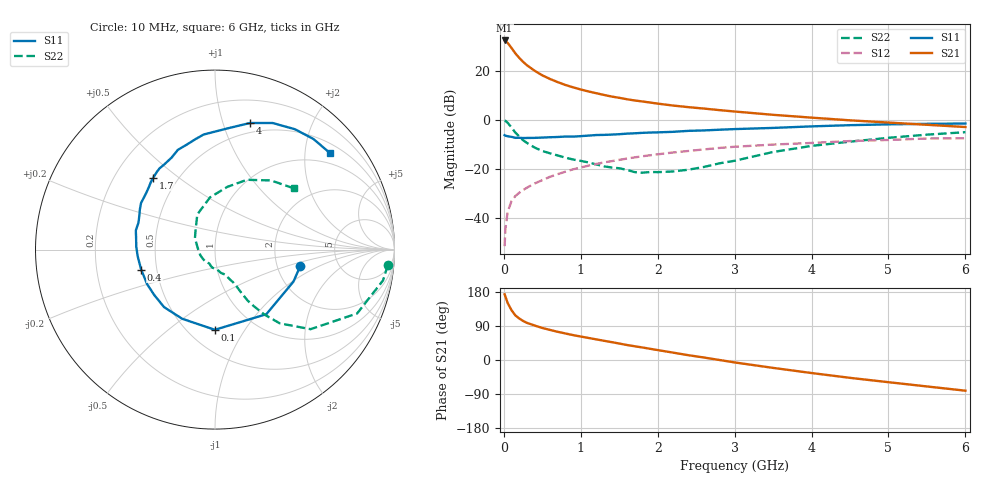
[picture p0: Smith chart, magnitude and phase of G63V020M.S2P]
! SIEMENS Small Signal Semiconductors
! BFG193
! Si NPN RF Bipolar Junction Transistor in SOT223
! VCE = 3 V  IC = 20 mA
! Common Emitter S-Parameters:  August  1996
# GHz  S  MA  R  50
!  f  S11  S21  S12  S22
! GHz  MAG  ANG  MAG  ANG  MAG  ANG  MAG  ANG
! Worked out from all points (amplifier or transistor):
!   36 points, 10 MHz to 6 GHz, reference 50 ohm
!   highest |S21| = 32.4 dB at 10 MHz (marker M1)
!   |S21| within 3 dB of that: start of sweep to 97.86 MHz
!   unconditionally stable (mu >= 1): 680.1 MHz to 2.463 GHz
!   at 250 MHz: K = 0.75, MSG = 26.2 dB, |S12| = -28.7 dB
!   at 1.4 GHz: K = 1.05, MAG = 11.8 dB, |S12| = -16.9 dB
!   at 6 GHz: K = 0.89, MSG = 2.3 dB, |S12| = -7.6 dB
!   S11 on the Smith chart (normalised r, x): 10 MHz: 2.69, -0.65; 100 MHz: 0.67, -0.74; 400 MHz: 0.41, -0.11; 1.7 GHz: 0.37, +0.41; 4 GHz: 0.41, +1.23; 6 GHz: 0.72, +2.59
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0.01  0.4834 -11.1  41.84 173.3  0.0026 89.5  0.9667 -5.2
0.02  0.4722 -22.1  41 167.8  0.0058 80.9  0.9517 -10.4
0.05  0.4599 -51.5  37.22 150.3  0.0131 72.0  0.8681 -24.2
0.1  0.4468 -90.1  29.32 131.4  0.0218 63.5  0.6927 -39.8
0.15  0.4265 -115.4  22.75 117.6  0.0276 58.2  0.5469 -48.7
0.2  0.428 -131.5  18.44 109.5  0.0321 57.9  0.4535 -52.8
0.25  0.4226 -143.2  15.28 103.1  0.0366 58.1  0.3811 -55.6
0.3  0.4244 -152.8  13.05 98.1  0.0408 59.1  0.3364 -57.4
0.4  0.4262 -164.9  10.05 91.0  0.0497 60.1  0.2702 -58.9
0.5  0.4323 -175.0  8.099 84.5  0.0583 60.0  0.2299 -59.8
0.6  0.439 177.9  6.823 79.4  0.0682 60.2  0.206 -61.2
0.7  0.4442 171.7  5.891 74.4  0.0772 59.7  0.1862 -63.4
0.9  0.4519 160.7  4.605 65.7  0.0969 57.5  0.154 -67.1
1.1  0.4739 152.1  3.791 58.2  0.115 55.0  0.1341 -75.7
1.4  0.4972 140.1  2.986 47.2  0.1422 49.7  0.1058 -90.6
1.7  0.5281 130.5  2.481 36.3  0.1702 44.1  0.085 -110.9
2.2  0.5665 115.3  1.953 19.5  0.2142 33.2  0.0876 -159.9
3.5  0.6811 83.6  1.262 -20.8  0.311 3.0  0.2191 116.8
4  0.732 74.5  1.105 -34.4  0.3355 -6.7  0.292 95.5
4.5  0.775 65.5  0.973 -47.1  0.3667 -16.8  0.3566 78.8
5.5  0.825 48.3  0.789 -69.8  0.4131 -40.2  0.4958 51.0
6  0.837 39.8  0.71 -81.0  0.4189 -53.7  0.5571 37.7
